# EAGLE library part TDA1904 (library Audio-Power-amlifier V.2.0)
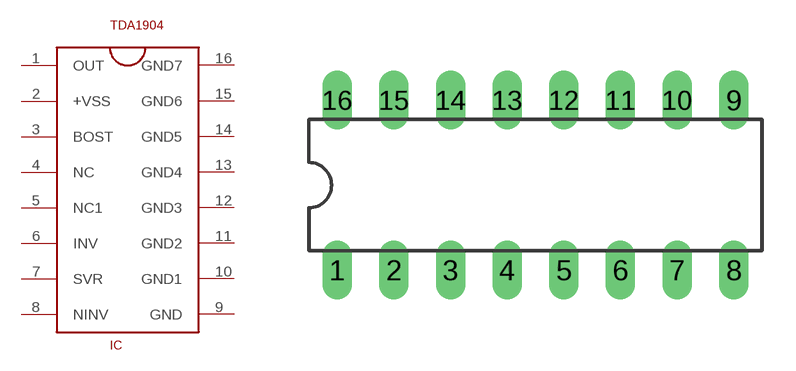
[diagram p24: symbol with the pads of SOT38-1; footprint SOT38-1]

Designator prefix IC

## TDA1904  [SOT38-1]
1  OUT  out
2  +VSS  pwr
3  BOST
4  NC  nc
5  NC1  nc
6  INV  in
7  SVR  in
8  NINV  in
9  GND  pwr
10  GND1  pwr
11  GND2  pwr
12  GND3  pwr
13  GND4  pwr
14  GND5  pwr
15  GND6  pwr
16  GND7  pwr

## Footprint SOT38-1 (pad centres in mm)
Dual In Line Package
drill 0.813 long: 1 -8.89,-3.81; 2 -6.35,-3.81; 3 -3.81,-3.81; 4 -1.27,-3.81; 5 1.27,-3.81; 6 3.81,-3.81; 7 6.35,-3.81; 8 8.89,-3.81; 9 8.89,3.81; 10 6.35,3.81; 11 3.81,3.81; 12 1.27,3.81; 13 -1.27,3.81; 14 -3.81,3.81; 15 -6.35,3.81; 16 -8.89,3.81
